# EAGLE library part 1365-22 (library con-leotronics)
DUAL ROW STRAIGHT HEADER 1364 SERIES. 1.27mm x 1.27mm. Without Fixing Post. SMT Source: http://www.leotronics.co.uk/Conexcon/Data%20Sheets/sec.%20A/1364ing.pdf
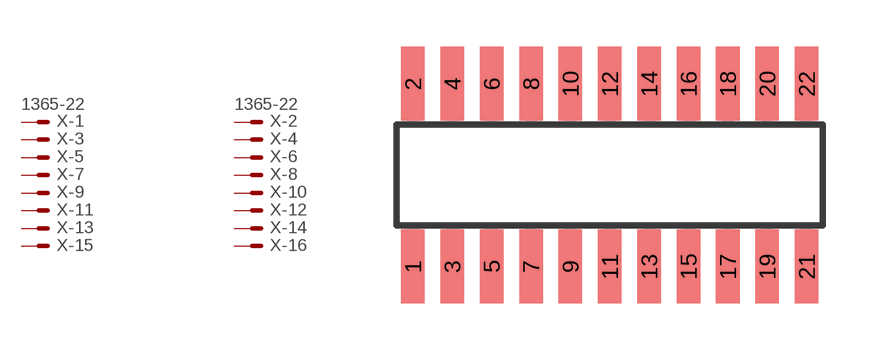
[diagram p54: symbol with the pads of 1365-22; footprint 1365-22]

Designator prefix X; gates -1=MVAL -2=MVAL -3=M -4=M -5=M -6=M -7=M -8=M -9=M -10=M -11=M -12=M -13=M -14=M -15=M -16=M -17=M -18=M -19=M -20=M -21=M -22=M

## 1365-22 (OC_FARNELL: unknown; OC_NEWARK: unknown)  [1365-22]
1  -1:S  pas
2  -2:S  pas
3  -3:S  pas
4  -4:S  pas
5  -5:S  pas
6  -6:S  pas
7  -7:S  pas
8  -8:S  pas
9  -9:S  pas
10  -10:S  pas
11  -11:S  pas
12  -12:S  pas
13  -13:S  pas
14  -14:S  pas
15  -15:S  pas
16  -16:S  pas
17  -17:S  pas
18  -18:S  pas
19  -19:S  pas
20  -20:S  pas
21  -21:S  pas
22  -22:S  pas

## Footprint 1365-22 (pad centres in mm)
DUAL ROW STRAIGHT HEADER 1364 SERIES. 1.27mm x 1.27mm. Without Fixing Post. SMT Source: http://www.leotronics.co.uk/Conexcon/Data%20Sheets/sec.%20A/1364ing.pdf
smd 0.76 x 2.4: 1 -6.35,-2.95; 2 -6.35,2.95; 3 -5.08,-2.95; 4 -5.08,2.95; 5 -3.81,-2.95; 6 -3.81,2.95; 7 -2.54,-2.95; 8 -2.54,2.95; 9 -1.27,-2.95; 10 -1.27,2.95; 11 0,-2.95; 12 0,2.95; 13 1.27,-2.95; 14 1.27,2.95; 15 2.54,-2.95; 16 2.54,2.95; 17 3.81,-2.95; 18 3.81,2.95; 19 5.08,-2.95; 20 5.08,2.95; 21 6.35,-2.95; 22 6.35,2.95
